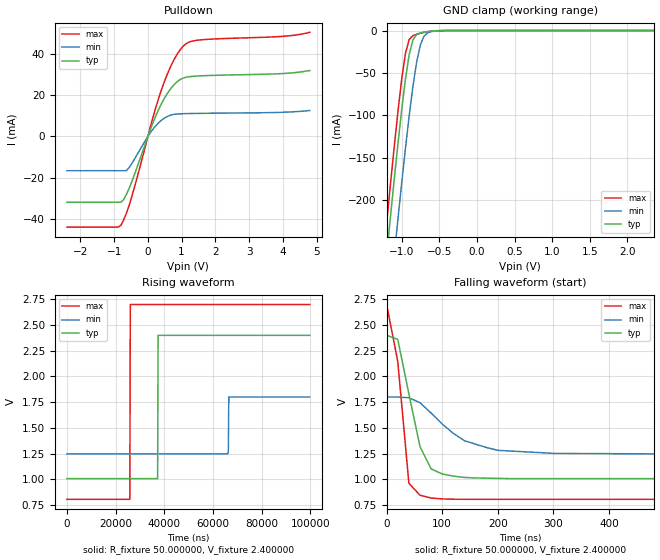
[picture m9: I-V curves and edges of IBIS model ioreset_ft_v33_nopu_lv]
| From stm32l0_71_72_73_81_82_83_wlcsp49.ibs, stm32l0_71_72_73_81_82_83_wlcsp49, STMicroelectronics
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|   Model ioreset_ft_v33_nopu_lv
[Model]  ioreset_ft_v33_nopu_lv
Model_type I/O_open_drain
Polarity   Inverting
Enable   Active-High
Vinl =   0.720000V
Vinh =   1.680000V
Vmeas =  1.200000V
Cref =   1.0000000000000001E-7F
Rref =   1.000000k
Vref =   2.400000V
C_comp   2.007500pF   1.959500pF   2.081200pF
[Temperature Range]   25.000000   0.125000k   -40.000000
[Pullup Reference]   2.400000V   1.800000V   2.700000V
[Pulldown Reference]   0.0V   0.0V   0.0V
[POWER Clamp Reference]   2.400000V   1.800000V   2.700000V
[GND Clamp Reference]   0.0V   0.0V   0.0V
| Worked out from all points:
|   slope of the pulldown table from 0 to 0.36 V, typ, clamps not added: 25 ohm
|   GND clamp passes 1 mA (typ) near -0.62 V on its own axis
|   rising waveform, R_fixture 50.000000, V_fixture 2.400000: 20-80 % time 120ns typ, 126ns min, 120ns max; typ from 1.01 V to 2.4 V
|   falling waveform, R_fixture 50.000000, V_fixture 2.400000: 20-80 % time 34ns typ, 79.4ns min, 22.6ns max; typ from 2.4 V to 1.01 V
[Pulldown]
|Voltage   I(typ)   I(min)   I(max)
-2.4V     -31.73mA   -16.51mA   -43.74mA
-880mV    -31.73mA   -16.51mA   -43.74mA
-800mV    -31.73mA   -16.51mA   -42.87mA
-640mV    -28.07mA   -16.51mA   -37.19mA
-480mV    -21.98mA   -13.17mA   -29.21mA
80mV      3.63mA     1.966mA    5.014mA
480mV     18.16mA    8.738mA    26.02mA
800mV     25.38mA    10.72mA    37.77mA
1.12V     28.53mA    11.02mA    44.6mA
1.6V      29.27mA    11.16mA    46.65mA
4V        30.36mA    11.67mA    48.3mA
4.8V      31.83mA    12.52mA    50.24mA
[GND_clamp]
|Voltage   I(typ)   I(min)   I(max)
-2.4V     -1.423A    -1.507A    -1.391A
-1.25V    -311.2mA   -401.9mA   -273.3mA
-1.2V     -265.4mA   -356.1mA   -227.2mA
-1.15V    -220.4mA   -310.8mA   -181.9mA
-1.1V     -176.3mA   -266.2mA   -137.9mA
-1.05V    -133.8mA   -222.5mA   -95.87mA
-950mV    -57.3mA    -138.9mA   -26.98mA
-900mV    -28.27mA   -100.4mA   -10.59mA
-850mV    -11.01mA   -65.54mA   -5.958mA
-750mV    -2.834mA   -16.5mA    -3.178mA
-600mV    -750uA     -1.164mA   -738.3uA
2.35V     0A         0A         0A
[POWER_clamp]
|Voltage   I(typ)   I(min)   I(max)
-2.4V     0A         0A         0A
0V        0A         0A         0A
[Ramp]
| variable   typ   min   max
dV/dt_r  0.83658/59.97419n   0.33204/60.33800n   1.13726/59.99367n
dV/dt_f  0.83652/62.01957n   0.33204/0.12819u   1.13726/60.11576n
R_load = 50.000000
[Rising Waveform]
R_fixture= 50.000000
V_fixture= 2.400000
V_fixture_min= 1.800000
V_fixture_max= 2.700000
|time   V(typ)   V(min)   V(max)
0s        1.006V     1.247V     804.6mV
25.83us   1.006V     1.247V     804.4mV
26.03us   1.006V     1.247V     2.7V
37.24us   1.006V     1.247V     2.7V
37.44us   2.4V       1.247V     2.7V
66.07us   2.4V       1.246V     2.7V
66.27us   2.4V       1.272V     2.7V
66.47us   2.4V       1.8V       2.7V
99.7us    2.4V       1.8V       2.7V
[Falling Waveform]
R_fixture= 50.000000
V_fixture= 2.400000
V_fixture_min= 1.800000
V_fixture_max= 2.700000
|time   V(typ)   V(min)   V(max)
0s        2.4V       1.8V       2.7V
20.02ns   2.361V     1.8V       2.146V
40.04ns   1.83V      1.793V     960.4mV
60.06ns   1.317V     1.745V     844.4mV
80.08ns   1.1V       1.643V     817.2mV
100.1ns   1.051V     1.536V     808.2mV
140.1ns   1.018V     1.374V     804.9mV
200.2ns   1.008V     1.281V     804.6mV
320.3ns   1.006V     1.251V     804.6mV
9.97us    1.006V     1.247V     804.6mV
